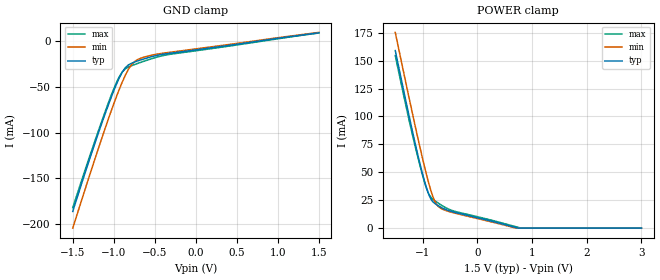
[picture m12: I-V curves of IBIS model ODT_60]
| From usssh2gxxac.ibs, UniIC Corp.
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|   Model ODT_60
[Model]  ODT_60
Model_type Input
Polarity   Non-Inverting
Vinl =   0.60000000V
Vinh =   0.90000000V
C_comp   1.6160pF   1.5990pF   1.6430pF
[Temperature Range]   25.0000   95.0000   0.0
[Voltage Range]   1.5000V   1.4000V   1.6000V
[GND_clamp]
|Voltage   I(typ)   I(min)   I(max)
-1.5V     -186.4mA   -204.7mA   -182.3mA
-1.22V    -109mA     -126.2mA   -106.6mA
-1.06V    -68.27mA   -83.56mA   -66mA
-980mV    -49.72mA   -63.56mA   -47.76mA
-940mV    -41.41mA   -54.16mA   -39.99mA
-900mV    -34.28mA   -45.34mA   -33.97mA
-860mV    -29mA      -37.33mA   -30.24mA
-780mV    -23.92mA   -25.21mA   -26.65mA
-740mV    -22.53mA   -21.73mA   -25.31mA
-580mV    -17.89mA   -16.1mA    -20.29mA
-340mV    -13.46mA   -12.35mA   -14.66mA
1.5V      9.293mA    9.746mA    9.055mA
[POWER_clamp]
|Voltage   I(typ)   I(min)   I(max)
-1.5V     159mA      175.3mA    154.6mA
-1.34V    121.7mA    138mA      117.5mA
-1.2V     89.9mA     105.9mA    86.52mA
-1.06V    59.91mA    74.87mA    58.28mA
-960mV    41.14mA    53.97mA    40.39mA
-900mV    31.87mA    42.41mA    32mA
-840mV    25.42mA    32.21mA    27.18mA
-780mV    22.19mA    24.37mA    24.65mA
-700mV    19.64mA    18.87mA    21.92mA
-440mV    14.46mA    13.79mA    15.49mA
749.7mV   0A         NA         NA
3V        0A         0A         0A
